[IBIS Ver]   4.0
[File name]   mpc5200b.ibs
[File Rev]   0.2
[Date]   April 07, 2005
[Source]   Freescale, TSPG, Transumer, DESIGN
[Notes]   IBIS model for the MPC5200B embedded microprocessor.
|   SDRAM (3.3V VDD_MEM) and DDR (2.5V VDD_MEM) configuration.
[Disclaimer]   This information is for modeling purposes only and
|   is not guaranteed.
[Copyright]   Copyright, Freescale, Inc., 2005
|   Component MPC5200B
[Component]   MPC5200B
[Manufacturer]   Freescale Inc.
[Package]
| variable   typ   min   max
R_pkg   100.0000m   NA   NA
L_pkg   6.0000nH   NA   NA
C_pkg   1.5000pF   NA   NA
[Pin] signal_name   model_name   R_pin   L_pin   C_pin
B02   test_mode_0   mdp12_4m   2.49E-01   1.06E-08   1.37E-12
A01   test_mode_1   mdp12_4m   2.06E-01   1.12E-08   1.46E-12
B01   test_sel_0   mdp12_4m   2.16E-01   1.21E-08   1.49E-12
C03   test_sel_1   mdp12_8m   1.88E-01   9.02E-09   1.44E-12
C02   rtc_xtal_in   NC   1.92E-01   9.53E-09   1.31E-12
C01   rtc_xtal_out   NC   2.05E-01   1.11E-08   1.29E-12
D03   timer2   mdp12_4m   1.89E-01   8.42E-09   1.25E-12
D02   timer3   mdp12_4m   2.02E-01   9.90E-09   1.29E-12
D04   vss_io   GND
D01   timer4   mdp12_4m   2.07E-01   1.08E-08   1.27E-12
D16   vss_core   GND
E03   timer5   mdp12_4m   1.96E-01   9.05E-09   1.22E-12
E02   timer6   mdp12_4m   2.03E-01   9.68E-09   1.24E-12
E01   timer7   mdp12_4m   2.08E-01   1.06E-08   1.28E-12
F03   usb1_9   mdp12_4m   1.93E-01   8.68E-09   1.21E-12
F02   usb1_8   mdp12_4m   1.98E-01   9.41E-09   1.19E-12
F01   usb1_7   mdp12_4m   2.03E-01   1.03E-08   1.22E-12
D06   vdd_io   POWER
G04   usb1_6   mdp12_4m   1.82E-01   7.65E-09   1.12E-12
G03   usb1_5   mdp12_4m   1.89E-01   8.37E-09   1.10E-12
G02   usb1_4   mdp12_4m   1.94E-01   9.11E-09   1.17E-12
D05   vdd_core   POWER
G01   usb1_3   mdp12_4m   2.01E-01   9.88E-09   1.15E-12
H03   usb1_2   mdp12_4m   1.83E-01   7.78E-09   1.04E-12
H02   usb1_1   mdp12_4m   1.90E-01   8.74E-09   1.13E-12
H01   usb1_0   mdp12_4m   1.97E-01   9.66E-09   1.10E-12
J04   eth_17   mdp12_4m   1.76E-01   7.04E-09   1.06E-12
J03   eth_10   mdp12_4m   1.81E-01   7.81E-09   1.06E-12
J02   eth_04   mdp12_4m   1.88E-01   8.72E-09   1.11E-12
J09   vss_io   GND
J01   eth_03   mdp12_4m   1.95E-01   9.39E-09   1.05E-12
K03   eth_02   mdp12_4m   1.80E-01   7.63E-09   1.05E-12
J10   vss_core   GND
K02   eth_01   mdp12_4m   1.86E-01   8.60E-09   1.09E-12
K01   eth_00   mdp12_4m   1.92E-01   9.30E-09   1.06E-12
L04   eth_11   mdp12g4m   1.74E-01   7.07E-09   1.04E-12
L03   eth_05   mdp12_4m   1.80E-01   7.87E-09   1.07E-12
L02   eth_16   mdp12_4m   1.87E-01   8.52E-09   1.06E-12
D09   vdd_io   POWER
L01   eth_09   mdp12g4m   1.94E-01   9.45E-09   1.10E-12
M03   eth_08   mdp12_4m   1.81E-01   7.91E-09   1.07E-12
M02   eth_12   mdp12_4m   1.89E-01   8.91E-09   1.11E-12
M01   eth_13   mdp12_4m   1.95E-01   9.76E-09   1.12E-12
N04   eth_14   mdp12_4m   1.79E-01   7.22E-09   1.01E-12
D07   vdd_core   POWER
N03   eth_15   mdp12_4m   1.82E-01   8.16E-09   1.09E-12
N02   eth_06   mdp12_4m   1.90E-01   9.03E-09   1.12E-12
N01   eth_07   mdp12_4m   1.96E-01   9.83E-09   1.16E-12
P03   irq_0   mdp12_4m   1.84E-01   8.33E-09   1.14E-12
P02   irq_2   mdp12_4m   1.91E-01   9.04E-09   1.12E-12
P01   irq_1   mdp12_4m   1.99E-01   9.99E-09   1.17E-12
J11   vss_io   GND
R04   pci_gnt_b   mdp12_8m   1.86E-01   8.03E-09   1.06E-12
R03   ext_ad_30   pci_33v   1.87E-01   8.62E-09   1.14E-12
E04   vdd_io   POWER
R02   pci_reset_b   pci_33v   1.94E-01   9.43E-09   1.23E-12
J12   vss_core   GND
R01   irq_3   mdp12_4m   2.01E-01   1.01E-08   1.28E-12
T03   ext_ad_28   pci_33v   1.89E-01   8.82E-09   1.25E-12
K09   vss_io   GND
T02   ext_ad_26   pci_33v   1.96E-01   9.63E-09   1.21E-12
T01   pci_clock   pci_33v   2.04E-01   1.07E-08   1.26E-12
F04   vdd_io   POWER
U03   ext_ad_24   pci_33v   1.96E-01   9.52E-09   1.30E-12
U02   pci_idsel   mdp12_8m   2.02E-01   1.01E-08   1.32E-12
D10   vdd_core   POWER
U01   pci_req_b   mdp12_8m   2.09E-01   1.10E-08   1.38E-12
V02   ext_ad_20   pci_33v   1.98E-01   1.03E-08   1.40E-12
K10   vss_io   GND
V01   ext_ad_31   pci_33v   2.07E-01   1.12E-08   1.40E-12
W01   ext_ad_29   pci_33v   2.03E-01   1.11E-08   1.44E-12
H04   vdd_io   POWER
Y01   ext_ad_27   pci_33v   2.12E-01   1.20E-08   1.43E-12
W02   ext_ad_25   pci_33v   1.98E-01   1.02E-08   1.39E-12
K11   vss_io   GND
Y02   pci_cbe_b_3   pci_33v   2.03E-01   1.09E-08   1.40E-12
V03   ext_ad_22   pci_33v   1.96E-01   9.75E-09   1.36E-12
T04   vdd_io   POWER
W03   ext_ad_23   pci_33v   1.99E-01   1.02E-08   1.30E-12
Y03   ext_ad_21   pci_33v   2.03E-01   1.09E-08   1.38E-12
K12   vss_io   GND
V04   ext_ad_18   pci_33v   1.87E-01   8.72E-09   1.26E-12
W04   ext_ad_16   pci_33v   1.96E-01   9.57E-09   1.24E-12
U05   vdd_io   POWER
Y04   ext_ad_19   pci_33v   2.02E-01   1.08E-08   1.26E-12
V05   pci_frame_b   pci_33v   1.86E-01   8.49E-09   1.19E-12
L09   vss_core   GND
W05   pci_trdy_b   pci_33v   2.11E-01   9.39E-09   1.19E-12
L10   vss_io   GND
Y05   ext_ad_17   pci_33v   1.99E-01   1.03E-08   1.20E-12
V06   pci_stop_b   pci_33v   1.87E-01   8.39E-09   1.12E-12
W06   pci_cbe_b_2   pci_33v   1.92E-01   8.96E-09   1.17E-12
U06   vdd_io   POWER
Y06   pci_irdy_b   pci_33v   1.99E-01   9.94E-09   1.21E-12
V07   pci_par   pci_33v   1.83E-01   8.01E-09   1.17E-12
W07   pci_devsel_b   pci_33v   1.91E-01   8.82E-09   1.15E-12
D11   vdd_core   POWER
Y07   pci_perr_b   pci_33v   1.97E-01   9.88E-09   1.17E-12
L11   vss_io   GND
U08   ext_ad_15   pci_33v   1.76E-01   7.00E-09   1.04E-12
V08   ext_ad_13   pci_33v   1.82E-01   7.86E-09   1.04E-12
U09   vdd_io   POWER
W08   pci_serr_b   pci_33v   1.88E-01   8.56E-09   1.08E-12
Y08   pci_cbe_b_1   pci_33v   1.95E-01   9.61E-09   1.10E-12
V09   ext_ad_11   pci_33v   1.80E-01   7.79E-09   1.04E-12
L12   vss_io   GND
W09   ext_ad_14   pci_33v   1.87E-01   8.73E-09   1.03E-12
M09   vss_core   GND
Y09   ext_ad_12   pci_33v   1.93E-01   9.09E-09   1.05E-12
U10   vdd_io   POWER
V10   ext_ad_09   pci_33v   1.78E-01   7.39E-09   1.04E-12
W10   pci_cbe_b_0   pci_33v   1.84E-01   8.21E-09   1.04E-12
M10   vss_io   GND
Y10   ext_ad_10   pci_33v   1.91E-01   9.14E-09   1.03E-12
U11   ext_ad_06   pci_33v   1.74E-01   7.07E-09   1.05E-12
U13   vdd_io   POWER
V11   ext_ad_04   pci_33v   1.78E-01   7.60E-09   1.06E-12
W11   ext_ad_08   pci_33v   1.85E-01   8.34E-09   1.06E-12
M11   vss_io   GND
Y11   ext_ad_07   pci_33v   1.91E-01   9.08E-09   1.04E-12
K04   vdd_core   POWER
V12   ext_ad_02   pci_33v   1.79E-01   7.64E-09   1.03E-12
U16   vdd_io   POWER
W12   ext_ad_05   pci_33v   1.87E-01   8.61E-09   1.08E-12
Y12   ext_ad_03   pci_33v   1.92E-01   9.16E-09   1.06E-12
M12   vss_io   GND
V13   ext_ad_00   pci_33v   1.80E-01   7.83E-09   1.09E-12
W13   ext_ad_01   pci_33v   1.88E-01   8.61E-09   1.10E-12
Y13   lp_ts_b   mdp12_8m   1.97E-01   9.75E-09   1.06E-12
U14   lp_ack_b   mdp12_8m   1.85E-01   7.82E-09   1.03E-12
V14   lp_ale_b   mdp12_8m   1.84E-01   8.26E-09   1.13E-12
U04   vss_core   GND
W14   csb_0   mdp12_8m   1.90E-01   8.80E-09   1.15E-12
Y14   csb_1   mdp12_8m   1.96E-01   9.54E-09   1.15E-12
V15   csb_2   mdp12_8m   1.84E-01   8.45E-09   1.16E-12
U17   vss_io   GND
W15   csb_3   mdp12_8m   1.90E-01   9.31E-09   1.16E-12
Y15   csb_4   mdp12_8m   1.98E-01   1.03E-08   1.18E-12
V16   csb_5   mdp12_8m   2.03E-01   9.15E-09   1.22E-12
W16   lp_rwb   mdp12_8m   1.95E-01   9.63E-09   1.27E-12
M04   vdd_core   POWER
Y16   ata_isolation   mdp12_8m   2.03E-01   1.06E-08   1.29E-12
V17   ata_drq   mdp12_8m   1.93E-01   9.36E-09   1.31E-12
W17   ata_iow_b   mdp12_8m   1.97E-01   1.01E-08   1.32E-12
Y17   ata_ior_b   mdp12_8m   2.07E-01   1.11E-08   1.35E-12
W18   ata_iochrdy   mdp12_8m   2.00E-01   1.05E-08   1.39E-12
Y18   ata_dack_b   mdp12_8m   2.09E-01   1.12E-08   1.40E-12
Y19   ata_intrq   mdp12_8m   2.13E-01   1.20E-08   1.47E-12
Y20   timer0   mdp12_4m   2.11E-01   1.22E-08   1.42E-12
W19   i2c1_io   mdp12g4m   2.01E-01   1.06E-08   1.43E-12
W20   i2c2_io   mdp12g4m   2.06E-01   1.12E-08   1.39E-12
V18   timer1   mdp12_4m   1.98E-01   1.01E-08   1.36E-12
V19   i2c1_clk   mdp12g4m   2.13E-01   1.18E-08   1.64E-12
V20   i2c2_clk   mdp12g4m   2.00E-01   1.06E-08   1.41E-12
U18   mem_mdq_31   mem_io   1.87E-01   8.83E-09   1.20E-12
U19   mem_mdq_01   mem_io   1.93E-01   9.71E-09   1.27E-12
U20   mem_mdq_00   mem_io   2.00E-01   1.07E-08   1.30E-12
D12   vdd_mem_io   POWER
T18   mem_mdq_30   mem_io   1.83E-01   8.41E-09   1.21E-12
T19   mem_mdq_03   mem_io   1.91E-01   9.36E-09   1.25E-12
T20   mem_mdq_02   mem_io   1.97E-01   1.03E-08   1.28E-12
R17   mem_mdq_28   mem_io   1.75E-01   7.52E-09   1.14E-12
R18   mem_mdq_29   mem_io   1.80E-01   8.10E-09   1.15E-12
R19   mem_mdq_05   mem_io   1.86E-01   8.81E-09   1.13E-12
D13   vdd_mem_io   POWER
R20   mem_mdq_04   mem_io   1.98E-01   1.00E-08   1.21E-12
P18   mem_mdq_27   mem_io   1.81E-01   7.96E-09   1.08E-12
P04   vdd_core   POWER
P19   mem_mdq_07   mem_io   1.89E-01   9.18E-09   1.12E-12
P20   mem_mdq_06   mem_io   1.97E-01   1.01E-08   1.20E-12
N17   mem_mdq_25   mem_io   1.60E-01   6.45E-09   1.02E-12
N18   mem_mdq_26   mem_io   1.80E-01   7.79E-09   1.08E-12
D15   vdd_mem_io   POWER
N19   mem_dqm_0   mem_io   1.88E-01   8.80E-09   1.12E-12
N20   mem_mdqs_0   mem_io   1.95E-01   9.71E-09   1.13E-12
M18   mem_mdq_24   mem_io   1.79E-01   7.71E-09   1.03E-12
M19   mem_mdq_14   mem_io   1.85E-01   8.61E-09   1.06E-12
M20   mem_mdq_15   mem_io   1.93E-01   9.59E-09   1.11E-12
L17   mem_dqm_3   mem_io   1.60E-01   6.40E-09   9.22E-13
D17   vdd_mem_io   POWER
L18   mem_mdqs_3   mem_io   1.79E-01   7.70E-09   1.06E-12
L19   mem_mdq_12   mem_io   1.86E-01   8.55E-09   1.06E-12
L20   mem_mdq_13   mem_io   1.92E-01   9.31E-09   1.08E-12
K18   mem_mdq_23   mem_io   1.80E-01   7.86E-09   1.06E-12
K19   mem_mdq_10   mem_io   1.87E-01   8.70E-09   1.09E-12
U07   vdd_core   POWER
K20   mem_mdq_11   mem_io   1.94E-01   9.44E-09   1.06E-12
E17   vdd_mem_io   POWER
J17   mem_mdq_22   mem_io   1.65E-01   6.76E-09   1.05E-12
J18   mem_mdq_21   mem_io   1.81E-01   8.11E-09   1.09E-12
J19   mem_mdq_08   mem_io   1.89E-01   9.00E-09   1.11E-12
J20   mem_mdq_09   mem_io   1.96E-01   9.73E-09   1.11E-12
H18   mem_mdq_20   mem_io   1.85E-01   8.42E-09   1.15E-12
H19   mem_dqm_1   mem_io   1.91E-01   9.14E-09   1.18E-12
F17   vdd_mem_io   POWER
H20   mem_mdqs_1   mem_io   1.98E-01   1.00E-08   1.18E-12
G17   mem_mdq_18   mem_io   1.84E-01   7.95E-09   1.10E-12
G18   mem_mdq_19   mem_io   1.86E-01   8.64E-09   1.18E-12
G19   mem_memclk   mem_io   1.93E-01   9.26E-09   1.19E-12
G20   mem_memclk_b   mem_io   2.00E-01   1.02E-08   1.23E-12
H17   vdd_mem_io   POWER
F18   mem_mdq_17   mem_io   1.95E-01   9.72E-09   1.27E-12
F19   mem_ma_12   mem_io   1.98E-01   9.92E-09   1.28E-12
U12   vdd_core   POWER
F20   mem_clk_en   mem_io   2.02E-01   1.04E-08   1.27E-12
E18   mem_mdq_16   mem_io   1.97E-01   9.41E-09   1.37E-12
E19   mem_ma_09   mem_io   1.95E-01   9.77E-09   1.28E-12
E20   mem_ma_11   mem_io   2.02E-01   1.08E-08   1.28E-12
K17   vdd_mem_io   POWER
D18   mem_mdqs_2   mem_io   1.98E-01   1.01E-08   1.37E-12
D19   mem_ma_07   mem_io   2.04E-01   1.04E-08   1.43E-12
D20   mem_ma_08   mem_io   2.12E-01   1.14E-08   1.47E-12
C20   mem_ma_06   mem_io   2.13E-01   1.17E-08   1.43E-12
C19   mem_ma_05   mem_io   2.09E-01   1.10E-08   1.45E-12
B20   mem_ma_04   mem_io   2.18E-01   1.22E-08   1.44E-12
M17   vdd_mem_io   POWER
A20   mem_dqm_2   mem_io   2.09E-01   1.18E-08   1.51E-12
B19   mem_cas_b   mem_io   2.08E-01   1.12E-08   1.47E-12
A19   mem_we_b   mem_io   2.19E-01   1.24E-08   1.49E-12
C18   mem_mba_0   mem_io   2.02E-01   9.98E-09   1.48E-12
B18   mem_cs0_b   mem_io   2.03E-01   1.07E-08   1.37E-12
A18   mem_ras_b   mem_io   2.10E-01   1.16E-08   1.37E-12
P17   vdd_mem_io   POWER
C17   mem_ma_00   mem_io   1.93E-01   9.24E-09   1.28E-12
B17   mem_ma_10   mem_io   2.00E-01   1.01E-08   1.28E-12
A17   mem_mba_1   mem_io   2.09E-01   1.08E-08   1.21E-12
C16   mem_ma_03   mem_io   1.87E-01   8.49E-09   1.21E-12
B16   mem_ma_02   mem_io   1.94E-01   9.44E-09   1.22E-12
U15   vdd_core   POWER
A16   mem_ma_01   mem_io   2.00E-01   1.01E-08   1.15E-12
C15   gpio_wkup_6   mem_io   1.82E-01   8.19E-09   1.04E-12
T17   vdd_mem_io   POWER
B15   clk_test_out   mdp12_4m   2.03E-01   9.96E-09   1.25E-12
A15   sys_xtal_in   NC   1.96E-01   1.02E-08   1.13E-12
D14   sys_xtal_out   NC   1.71E-01   7.02E-09   1.16E-12
C14   sys_pll_avss   GND
B14   sys_pll_avdd   POWER
A14   sreset_b   mdp12g8m   1.99E-01   9.63E-09   1.09E-12
C13   ir_usb_clk   mdp12_4m   1.85E-01   8.10E-09   1.10E-12
B13   hreset_b   mdp12g8m   1.91E-01   8.85E-09   1.07E-12
A13   porreset_b   mdp12g4m   1.97E-01   9.42E-09   1.07E-12
C12   gpio_wkup_7   mdp12_8m   2.08E-01   7.88E-09   1.03E-12
B12   ir_rx   mdp12_4m   1.88E-01   8.59E-09   1.08E-12
A12   ir_tx   mdp12_4m   1.95E-01   9.35E-09   1.09E-12
C11   irda_rx   mdp12_4m   1.81E-01   7.89E-09   1.07E-12
B11   psc1_0   mdp12_4m   1.89E-01   8.71E-09   1.07E-12
A11   psc1_1   mdp12_4m   1.95E-01   9.65E-09   1.11E-12
C10   psc1_2   mdp12_4m   1.83E-01   8.17E-09   1.08E-12
B10   psc1_3   mdp12_4m   1.89E-01   8.95E-09   1.12E-12
A10   psc1_4   mdp12_4m   1.95E-01   9.67E-09   1.11E-12
C09   psc2_0   mdp12_4m   1.83E-01   8.26E-09   1.10E-12
B09   psc2_1   mdp12_4m   1.90E-01   9.19E-09   1.10E-12
A09   psc2_2   mdp12_4m   1.96E-01   9.89E-09   1.10E-12
D08   lp_oe_b   mdp12_8m   1.85E-01   8.06E-09   1.02E-12
C08   harpo_pll_avdd  POWER
B08   psc2_3   mdp12_4m   1.89E-01   9.02E-09   1.12E-12
A08   psc2_4   mdp12_4m   1.96E-01   9.93E-09   1.09E-12
C07   psc3_0   mdp12_4m   1.85E-01   8.41E-09   1.14E-12
B07   psc3_1   mdp12_4m   1.92E-01   9.14E-09   1.17E-12
A07   psc3_2   mdp12_4m   1.98E-01   9.96E-09   1.16E-12
C06   psc3_3   mdp12_4m   1.88E-01   8.80E-09   1.16E-12
B06   psc3_4   mdp12_4m   1.93E-01   9.50E-09   1.19E-12
A06   psc3_5   mdp12_4m   1.97E-01   1.01E-08   1.21E-12
C05   psc3_6   mdp12_4m   1.89E-01   8.87E-09   1.24E-12
B05   psc3_7   mdp12_4m   1.95E-01   9.78E-09   1.25E-12
A05   psc3_8   mdp12_4m   2.03E-01   1.08E-08   1.31E-12
C04   psc3_9   mdp12_4m   1.90E-01   9.24E-09   1.29E-12
B04   jtag_tck   mdp12_4m   1.99E-01   1.03E-08   1.32E-12
A04   jtag_tms   mdp12_4m   2.05E-01   1.10E-08   1.27E-12
A03   jtag_tdi   mdp12_4m   2.37E-01   1.11E-08   1.34E-12
B03   jtag_trst_b   mdp12_4m   1.95E-01   9.85E-09   1.36E-12
A02   jtag_tdo   mdp12_8m   2.12E-01   1.17E-08   1.45E-12
[Model Selector]   mem_io
mdp25v16   I/O for DDR configuration (2.5V VDD_MEM)
mdp33v16   I/O for SDR configuration (3.3V VDD_MEM)
| Models and submodels in the file (7): mdp25v16 (I/O), mdp33v16 (I/O), mdp12_4m (I/O), mdp12_8m (I/O), mdp12g4m (I/O), mdp12g8m (I/O), pci_33v (I/O)
